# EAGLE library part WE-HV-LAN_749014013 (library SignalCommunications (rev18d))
WE-LAN HV LAN-Transformer Characteristics: •Compliant with IEEE802.3 and 802.3af standards •Operating temperature: 0 °C to +70 °C •SMD •4 kV Hipot test Applications: •Ethernet •Compliant with most IC's for Ethernet applications like Intel, AMD, Conexant, Realtek, etc. •Hub, Router, Switches, medical applications Details see: http://katalog.we-online.de/en/pbs/WE-LAN/749014013 Updated by Dan Xu 2014-07-08 2014 (C) Würth Elektronik
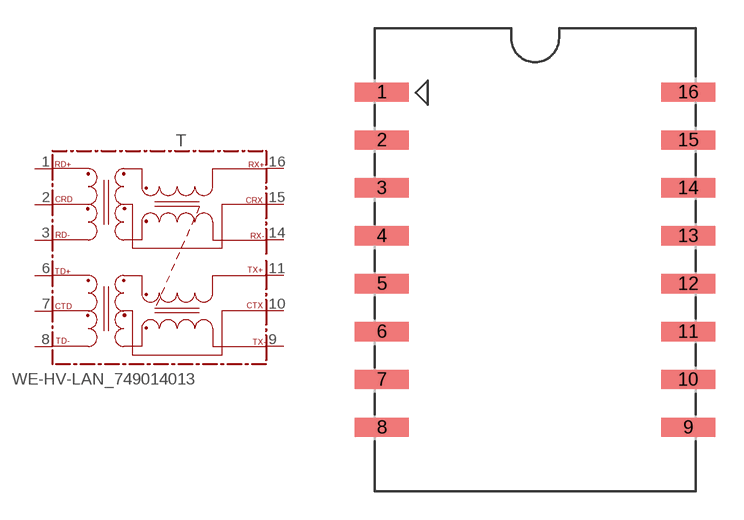
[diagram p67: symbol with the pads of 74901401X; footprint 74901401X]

Designator prefix T

## WE-HV-LAN_749014013  [74901401X]
1  RD+
2  CRD
3  RD-
6  TD+
7  CTD
8  TD-
9  TX-
10  CTX
11  TX+
14  RX-
15  CRX
16  RX+

## Footprint 74901401X (pad centres in mm)
MAX Height=10.85 mm
smd 2.87 x 1.02: 1 -8.115,8.89; 2 -8.115,6.35; 3 -8.115,3.81; 4 -8.115,1.27; 5 -8.115,-1.27; 6 -8.115,-3.81; 7 -8.115,-6.35; 8 -8.115,-8.89; 9 8.115,-8.89; 10 8.115,-6.35; 11 8.115,-3.81; 12 8.115,-1.27; 13 8.115,1.27; 14 8.115,3.81; 15 8.115,6.35; 16 8.115,8.89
